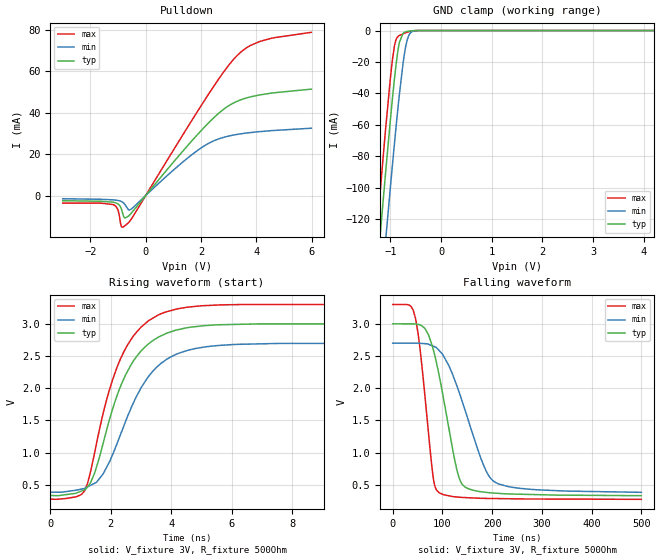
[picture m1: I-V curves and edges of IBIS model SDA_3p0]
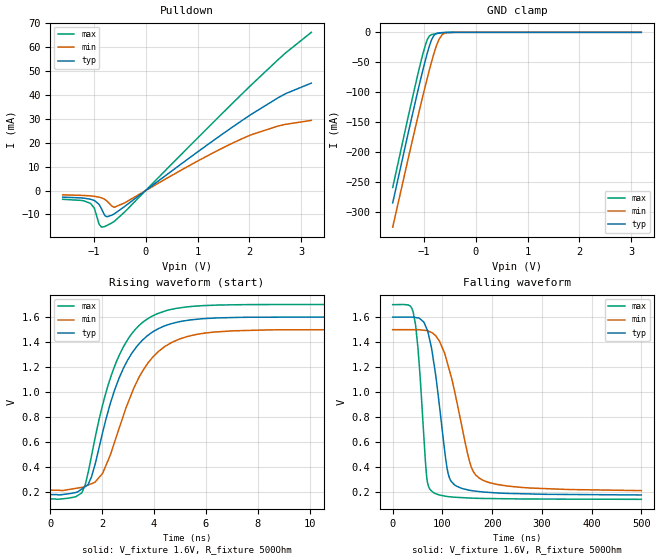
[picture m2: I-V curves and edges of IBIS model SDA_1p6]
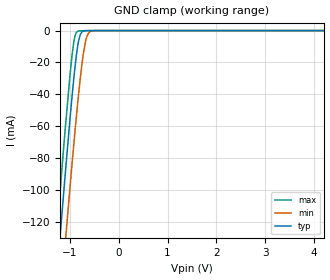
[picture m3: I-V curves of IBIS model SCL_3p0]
|Texas Instruments Incorporated
| 4 W Class-D Mono Audio Amplifier with Class-G Boost and Speaker Sense
| Marketing part#   Digital Voltage Range   Package-type   #pins
| TAS2552   1.5V-3.3V   WCSP   30
[IBIS Ver]   4.1
[File name]   tas2552.ibs
[File Rev]   1.0
[Date]   02/07/2014
[Source]
| Texas Instruments Incorporated.
| Analog-eLab Design Center, HPA
| 12500 TI Blvd
| Dallas, TX -75243
[Notes]   Revision History:
| Rev 1.0: 02/07/2014
| - Initial version of the model
| - Model generated from simulations in TISPICE
| - C_comp although listed in numerical order of value are
|   obtained from varying PVT conditions. For PVT conditions for
|   each specific value refer the buffer description under
|   respective [Model]. IBIS model user is responsible for using
|   appropriate C_comp to simulate for Signal Integrity.
| - Warnings regarding combined Non-monotonicity of various models have been
|   reviewd and considered minor and can be ignored.
| - Model names with a trailing _1p6 contains the model for lower Vcc range.
|   Model names with a trailing _3p0 contains the model
|   for higher Vcc range.
[Disclaimer]
| This model is designed as an aid for customers of Texas Instruments.
| TI and its licensors and suppliers make no warranties, either expressed
| or implied, with respect to this  model, including the warranties of
| merchantability or fitness for a particular purpose. The model is
| provided solely on an "as is" basis. The entire risk as to its quality
| and performance is with the customer.
[Copyright]
 (C) Copyright 2014 Texas Instruments Incorporated.All rights reserved.
|   TAS2552
[Component]   TAS2552
[Manufacturer]   TI
[Package]   | 36 pin LLP
| variable   typ   min   max
R_pkg   0.01   0.008   0.12
L_pkg   0.1nH   0.08nH   0.12nH
C_pkg   0.1pF   0.08pF   0.12pF
[Pin]  signal_name   model_name   R_pin   L_pin   C_pin
A1   PGND   GND   NA   NA   NA
A2   OUT-   NC   NA   NA   NA
A3   OUT+   NC   NA   NA   NA
A4   PVDD   POWER   NA   NA   NA
A5   VBOOST   NC   NA   NA   NA
B1   BIAS   NC   NA   NA   NA
B2   VSENSE-   NC   NA   NA   NA
B3   VSENSE+   NC   NA   NA   NA
B4   SW   NC   NA   NA   NA
B5   SW   NC   NA   NA   NA
C1   AGND   GND   NA   NA   NA
C2   AGND   GND   NA   NA   NA
C3   VREG   NC   NA   NA   NA
C4   PGND   GND   NA   NA   NA
C5   PGND   GND   NA   NA   NA
D1   VBAT   NC   NA   NA   NA
D2   AIN-   NC   NA   NA   NA
D3   DIN   MCLK   NA   NA   NA
D4   ADDR   MCLK   NA   NA   NA
D5   SDA   SDA   NA   NA   NA
E1   AVDD   POWER   NA   NA   NA
E2   AIN+   NC   NA   NA   NA
E3   DOUT   DOUT   NA   NA   NA
E4   IVCLKIN   SCL   NA   NA   NA
E5   SCL   SCL   NA   NA   NA
F1   IOVDD   POWER   NA   NA   NA
F2   EN   MCLK   NA   NA   NA
F3   WCLK   BCLK   NA   NA   NA
F4   BCLK   BCLK   NA   NA   NA
F5   MCLK   MCLK   NA   NA   NA
|   Model Selectors
[Model Selector]  MCLK
MCLK_3p0   Input buffer in higher power supply range
MCLK_1p6   Input buffer in lower power supply range
[Model Selector]  SCL
SCL_3p0   SCL buffer in higher power supply range
SCL_1p6   SCL buffer in lower power supply range
[Model Selector]  BCLK
BCLK_3p0   BCLK buffer in higher power supply range
BCLK_1p6   BCLK buffer in lower power supply range
[Model Selector]  SDA
SDA_3p0   BCLK buffer in higher power supply range
SDA_1p6   BCLK buffer in lower power supply range
[Model Selector]  DOUT
DOUT_3p0   BCLK buffer in higher power supply range
DOUT_1p6   BCLK buffer in lower power supply range
| Models and submodels in the file (10): SDA_3p0 (I/O_open_drain), SDA_1p6 (I/O_open_drain), SCL_3p0 (Input), SCL_1p6 (Input), MCLK_3p0 (Input), MCLK_1p6 (Input), DOUT_3p0 (Output), DOUT_1p6 (Output), BCLK_3p0 (I/O), BCLK_1p6 (I/O)
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|   Model
[Model]   SDA_3p0
Model_type   I/O_open_drain
Polarity   Non-Inverting
Enable   Active-Low
Vinl = 0.9
Vinh = 2.1
Vmeas = 1.5
Vref = 0
Cref = 1pF
Rref = 1000000
|   typ   min   max
C_comp   1.431pF   1.410pF   1.451pF
[Voltage Range]   3   2.7   3.3
[Temperature Range]   27   125   -40
[Pullup Reference]   3   2.7   3.3
[Pulldown Reference]   -0   -0   -0
[Power Clamp Reference]   3   2.7   3.3
[GND Clamp Reference]   -0   -0   -0
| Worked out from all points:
|   slope of the pulldown table from 0 to 0.45 V, typ, clamps not added: 61.5 ohm
|   GND clamp passes 1 mA (typ) near -0.71 V on its own axis
|   falling waveform, V_fixture 3V, R_fixture 500Ohm: 20-80 % time 39.4ns typ, 61.3ns min, 23.8ns max; typ from 3 V to 0.332 V
|   rising waveform, V_fixture 3V, R_fixture 500Ohm: 20-80 % time 1.23ns typ, 1.39ns min, 1.17ns max; typ from 0.332 V to 3 V
[Pulldown]
|   Voltage   I(typ)   I(min)   I(max)
-3V       -2.494mA   -1.536mA   -3.627mA
-1.173V   -3.222mA   -2.079mA   -4.386mA
-1.002V   -4.047mA   -2.375mA   -6.915mA
-930mV    -5.029mA   -2.61mA    -11.58mA
-876mV    -6.557mA   -2.884mA   -14.93mA
-795mV    -10.15mA   -3.609mA   -15.03mA
-525mV    -8.576mA   -6.573mA   -11.49mA
1.896V    29.79mA    22mA       41.13mA
2.67V     40.11mA    27.52mA    56.9mA
3.282V    45.41mA    29.5mA     67.32mA
4.119V    48.63mA    30.9mA     74.45mA
5.991V    51.44mA    32.55mA    78.9mA
[GND Clamp]
|   Voltage   I(typ)   I(min)   I(max)
-3V       -845mA     -876.8mA   -826mA
-1.335V   -181.2mA   -223.5mA   -154mA
-1.173V   -119.4mA   -162.6mA   -91.63mA
-1.092V   -89.4mA    -132.7mA   -61.67mA
-993mV    -54.33mA   -97.12mA   -28.09mA
-912mV    -28.4mA    -69.19mA   -8.545mA
-867mV    -16.33mA   -54.42mA   -4.432mA
-822mV    -7.485mA   -40.46mA   -3.149mA
-714mV    -1mA       -13.1mA    -1.639mA
-624mV    -307uA     -2.395mA   -703.4uA
-489mV    -22.33uA   -84.56uA   -58.75uA
5.991V    0A         0A         0A
[POWER Clamp]
|   Voltage   I(typ)   I(min)   I(max)
-3V       0A         0A         0A
-2.982V   0A         0A         0A
-2.973V   0A         0A         0A
5.991V    0A         0A         0A
[Ramp]
R_load = 500
|   typ   min   max
dV/dt_r   1.60094/1.22524e-09   1.38987/1.39405e-09   1.81483/1.16909e-09
dV/dt_f   1.60093/3.93622e-08   1.38987/6.12483e-08   1.81483/2.37949e-08
[Falling Waveform]
V_fixture = 3V
V_fixture_min = 2.7V
V_fixture_max = 3.3V
R_fixture = 500Ohm
C_fixture = 0F
|   Time   V(typ)   V(min)   V(max)
0s        3V         2.7V       3.3V
45.93ns   2.997V     2.7V       3.084V
56.03ns   2.981V     2.697V     2.538V
80.72ns   2.626V     2.655V     658.5mV
92.41ns   2.234V     2.593V     383.8mV
128.8ns   742.3mV    2.042V     311.8mV
144.8ns   470.2mV    1.677V     302.9mV
183.9ns   386.7mV    784.1mV    290.1mV
210.6ns   368.8mV    521.7mV    287mV
500ns     331.8mV    383.6mV    275.3mV
[Rising Waveform]
V_fixture = 3V
V_fixture_min = 2.7V
V_fixture_max = 3.3V
R_fixture = 500Ohm
C_fixture = 0F
|   Time   V(typ)   V(min)   V(max)
0s        331.8mV    383.6mV    275.3mV
1.129ns   420.9mV    441.7mV    400.1mV
1.468ns   685.1mV    523.1mV    1.006V
2.058ns   1.675V     966.6mV    2.13V
2.488ns   2.206V     1.483V     2.617V
2.991ns   2.574V     1.999V     2.945V
3.513ns   2.776V     2.325V     3.123V
4.167ns   2.903V     2.528V     3.229V
6.389ns   2.994V     2.683V     3.3V
500ns     3V         2.7V       3.3V
|   Model
[Model]   SDA_1p6
Model_type   I/O_open_drain
Polarity   Non-Inverting
Enable   Active-Low
Vinl = 0.48
Vinh = 1.12
Vmeas = 0.8
Vref = 0
Cref = 1pF
Rref = 1000000
|   typ   min   max
C_comp   1.431pF   1.410pF   1.451pF
[Voltage Range]   1.6   1.5   1.7
[Temperature Range]   27   125   -40
[Pullup Reference]   1.6   1.5   1.7
[Pulldown Reference]   -0   -0   -0
[Power Clamp Reference]   1.6   1.5   1.7
[GND Clamp Reference]   -0   -0   -0
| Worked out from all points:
|   slope of the pulldown table from 0 to 0.24 V, typ, clamps not added: 61.3 ohm
|   GND clamp passes 1 mA (typ) near -0.71 V on its own axis
|   falling waveform, V_fixture 1.6V, R_fixture 500Ohm: 20-80 % time 27.2ns typ, 43.8ns min, 15.8ns max; typ from 1.6 V to 0.176 V
|   rising waveform, V_fixture 1.6V, R_fixture 500Ohm: 20-80 % time 1.39ns typ, 1.54ns min, 1.34ns max; typ from 0.176 V to 1.6 V
[Pulldown]
|   Voltage   I(typ)   I(min)   I(max)
-1.6V     -2.757mA   -1.805mA   -3.66mA
-1.067V   -3.602mA   -2.233mA   -5.331mA
-990.4mV  -4.16mA    -2.406mA   -7.4mA
-899.2mV  -5.781mA   -2.753mA   -13.95mA
-851.2mV  -7.622mA   -3.055mA   -15.27mA
-750.4mV  -10.91mA   -4.303mA   -14.62mA
-620.8mV  -9.924mA   -6.868mA   -13.09mA
-400mV    -6.565mA   -5.094mA   -8.844mA
948.8mV   15.29mA    11.67mA    20.78mA
1.904V    29.91mA    22.07mA    41.3mA
2.672V    40.13mA    27.53mA    56.94mA
3.195V    44.86mA    29.3mA     66.07mA
[GND Clamp]
|   Voltage   I(typ)   I(min)   I(max)
-1.6V     -284.6mA   -325.2mA   -258.9mA
-1.134V   -105mA     -148.2mA   -77.17mA
-1.014V   -61.68mA   -104.7mA   -34.84mA
-956.8mV  -42.27mA   -84.45mA   -17.81mA
-894.4mV  -23.38mA   -63.32mA   -6.363mA
-841.6mV  -10.84mA   -46.4mA    -3.565mA
-808mV    -5.607mA   -36.32mA   -2.909mA
-707.2mV  -913.8uA   -11.83mA   -1.559mA
-640mV    -385.5uA   -3.407mA   -845.9uA
-568mV    -120.5uA   -634uA     -311.8uA
-400mV    -2.227uA   -8.377uA   -4.851uA
3.195V    0A         0A         0A
[POWER Clamp]
|   Voltage   I(typ)   I(min)   I(max)
-1.6V     0A         0A         0A
-1.59V    0A         0A         0A
-1.586V   0A         0A         0A
3.195V    0A         0A         0A
[Ramp]
R_load = 500
|   typ   min   max
dV/dt_r   0.854214/1.3867e-09   0.773193/1.54211e-09   0.935047/1.33965e-09
dV/dt_f   0.854211/2.71793e-08   0.773193/4.36564e-08   0.935049/1.58159e-08
[Falling Waveform]
V_fixture = 1.6V
V_fixture_min = 1.5V
V_fixture_max = 1.7V
R_fixture = 500Ohm
C_fixture = 0F
|   Time   V(typ)   V(min)   V(max)
0s        1.6V       1.5V       1.7V
41.1ns    1.6V       1.5V       1.643V
50.71ns   1.594V     1.5V       1.356V
68.42ns   1.507V     1.492V     319.9mV
80.17ns   1.299V     1.473V     200.8mV
109.6ns   386.5mV    1.239V     164.5mV
126.1ns   252.7mV    976.8mV    158.1mV
156.7ns   212.4mV    416.1mV    151.5mV
180.8ns   200.5mV    295.9mV    148.7mV
500ns     176.3mV    211.3mV    141.6mV
[Rising Waveform]
V_fixture = 1.6V
V_fixture_min = 1.5V
V_fixture_max = 1.7V
R_fixture = 500Ohm
C_fixture = 0F
|   Time   V(typ)   V(min)   V(max)
0s        176.3mV    211.3mV    141.6mV
1.219ns   221.4mV    234.3mV    190.3mV
1.592ns   319mV      263.5mV    488.3mV
2.017ns   671.7mV    345.8mV    893.8mV
2.334ns   918.6mV    505mV      1.121V
2.811ns   1.185V     804.2mV    1.357V
3.283ns   1.349V     1.056V     1.502V
4.429ns   1.53V      1.365V     1.649V
6.565ns   1.594V     1.483V     1.697V
500ns     1.6V       1.5V       1.7V
|   Model
[Model]   SCL_3p0
Model_type   Input
Vinl = 0.9
Vinh = 2.1
|   typ   min   max
C_comp   1.010pF   0.982pF   1.067pF
[Voltage Range]   3   2.7   3.3
[Temperature Range]   27   125   -40
[Power Clamp Reference]   3   2.7   3.3
[GND Clamp Reference]   -0   -0   -0
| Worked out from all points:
|   GND clamp passes 1 mA (typ) near -0.76 V on its own axis
[GND Clamp]
|   Voltage   I(typ)   I(min)   I(max)
-3V       -843.1mA   -874.9mA   -823.7mA
-1.335V   -180.3mA   -222.6mA   -152.7mA
-1.173V   -118.6mA   -161.8mA   -90.27mA
-1.092V   -88.63mA   -131.9mA   -60.23mA
-957mV    -41.53mA   -83.83mA   -15.75mA
-894mV    -22.36mA   -62.51mA   -3.256mA
-840mV    -9.459mA   -45.24mA   -464.6uA
-786mV    -2.352mA   -29.44mA   -154uA
-696mV    -124.1uA   -9.252mA   -73.5uA
-633mV    -25uA      -2.445mA   -39.45uA
-552mV    -4.606uA   -280.5uA   -11.43uA
5.991V    0A         0A         0A
[POWER Clamp]
|   Voltage   I(typ)   I(min)   I(max)
-3V       0A         0A         0A
-2.982V   0A         0A         0A
-2.973V   0A         0A         0A
5.991V    0A         0A         0A
